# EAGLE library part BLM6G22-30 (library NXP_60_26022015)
W-CDMA 2100 MHz to 2200 MHz power MMIC 30 W LDMOS 2-stage power MMIC for base station applications at frequencies from 2100 MHz to 2200 MHz. Available in gull wing for surface mount (!SOT822-1!) or flat lead (SOT834-1). AAL Eindhoven MK
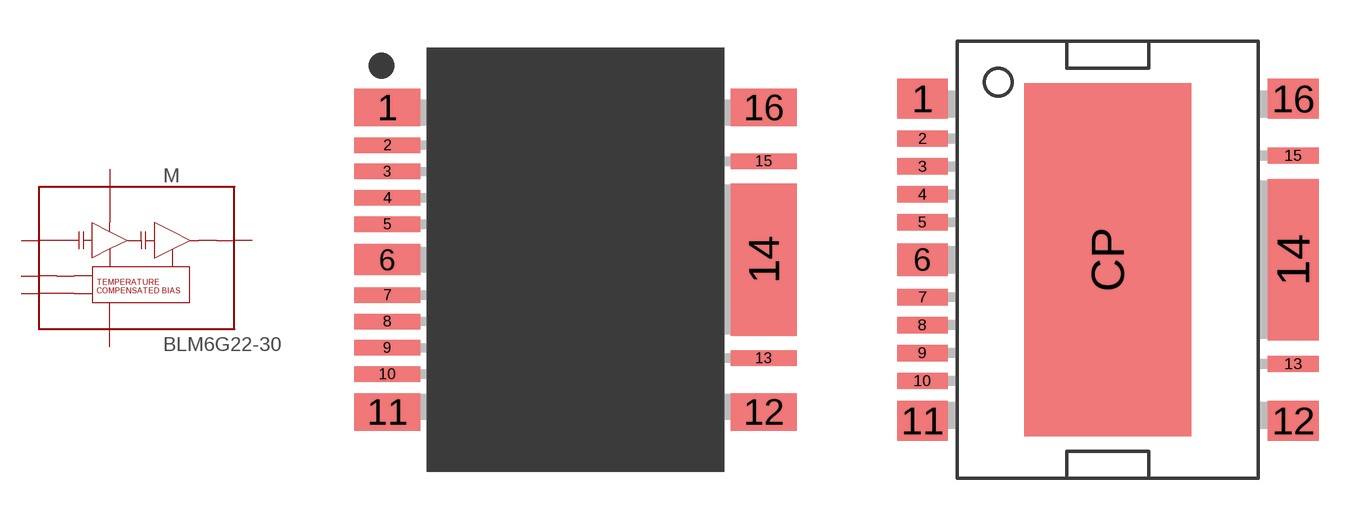
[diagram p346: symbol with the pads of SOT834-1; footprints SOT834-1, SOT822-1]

Designator prefix M

## BLM6G22-30  [SOT834-1]
1  GND  pwr
2  VDS1  pwr
6  RFIN  in
9  VGS1  pas
10  VGS2  pas
11  GND  pwr
12  GND  pwr
14  RFOUT  out
16  GND  pwr

## BLM6G22-30G  [SOT822-1]
1  GND  pwr
2  VDS1  pwr
6  RFIN  in
9  VGS1  pas
10  VGS2  pas
11  GND  pwr
12  GND  pwr
14  RFOUT  out
16  GND  pwr
CP  GND  pwr

## Footprint SOT834-1 (pad centres in mm)
SOT834-1 HSOP16F: plastic, heatsink small outline package; 16 leads (flat) JEDEC: -- IEC: -- JEITA: --date: 2013-02-07
smd 2.55 x 1.45: 1 -7.275,5.89; 11 -7.275,-5.89; 12 7.275,-5.89; 16 7.275,5.89
smd 2.55 x 0.6: 2 -7.275,4.43; 3 -7.275,3.41; 4 -7.275,2.39; 5 -7.275,1.37; 7 -7.275,-1.37; 8 -7.275,-2.39; 9 -7.275,-3.41; 10 -7.275,-4.43; 13 7.275,-3.81; 15 7.275,3.81
smd 2.55 x 1.2: 6 -7.275,0
smd 2.55 x 5.9: 14 7.275,0

## Footprint SOT822-1 (pad centres in mm)
SOT822-1 HSOP16: plastic, heatsink small outline package; 16 leads JEDEC: -- IEC: -- JEITA: --date: 2013-02-08
smd 1.85 x 1.45: 1 -6.775,5.89; 11 -6.775,-5.89; 12 6.775,-5.89; 16 6.775,5.89
smd 1.85 x 0.6: 2 -6.775,4.43; 3 -6.775,3.41; 4 -6.775,2.39; 5 -6.775,1.37; 7 -6.775,-1.37; 8 -6.775,-2.39; 9 -6.775,-3.41; 10 -6.775,-4.43; 13 6.775,-3.81; 15 6.775,3.81
smd 1.85 x 1.2: 6 -6.775,0
smd 1.85 x 5.9: 14 6.775,0
smd 6.1 x 12.9: CP 0,0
